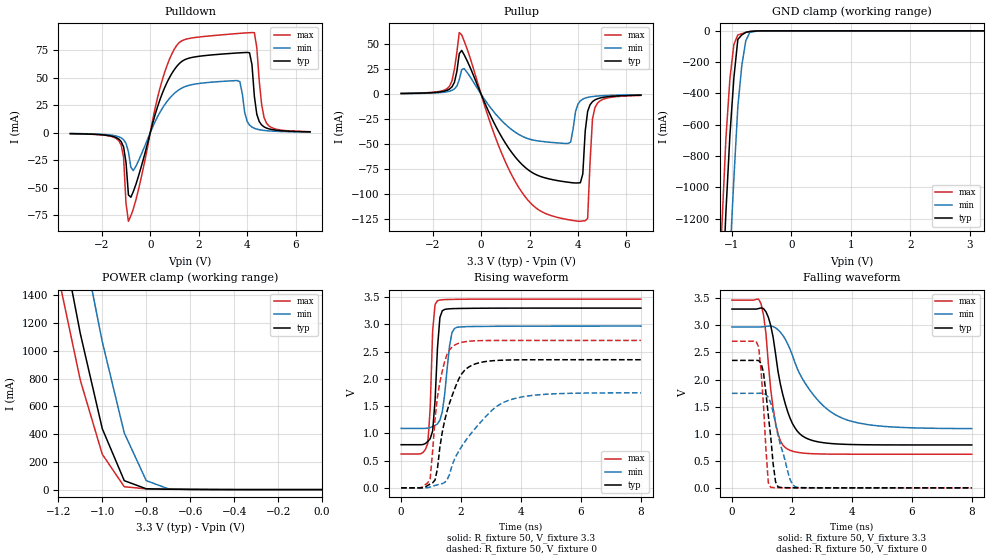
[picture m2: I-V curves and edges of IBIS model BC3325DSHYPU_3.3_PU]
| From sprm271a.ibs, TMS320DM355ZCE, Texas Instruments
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|   Component BC3325DSHYPU
|   Model Cell BC3325DSHYPU_3.3_PU
[Model]   BC3325DSHYPU_3.3_PU
Model_type   I/O
Polarity   Non-Inverting
Enable   Active-Low
Vinl =  1.5
Vinh =  1.8
Cref =  15.0000pF
Rref =  100.0000M
Vref =  0V
Vmeas =  1.65
C_comp   0.972592p   0.9599789p   0.9808023p
[Model Spec]
Vinl   1.5   1.335   1.5825
Vinh   1.8   1.635   1.8825
[Temperature Range]   25   125   -40
[Voltage Range]   3.3   2.97   3.465
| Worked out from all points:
|   slope of the pulldown table from 0 to 0.495 V, typ, clamps not added: 13.9 ohm
|   slope of the pullup table from 0 to 0.495 V, typ, clamps not added: 18.5 ohm
|   GND clamp passes 1 mA (typ) near -0.58 V on its own axis
|   POWER clamp passes 1 mA (typ) near -0.55 V on its own axis
|   rising waveform, R_fixture 50, V_fixture 3.3: 20-80 % time 158ps typ, 222ps min, 119ps max; typ from 0.792 V to 3.3 V
|   rising waveform, R_fixture 50, V_fixture 0: 20-80 % time 596ps typ, 1.31ns min, 352ps max; typ from 0.001 V to 2.35 V
|   falling waveform, R_fixture 50, V_fixture 3.3: 20-80 % time 567ps typ, 1.23ns min, 334ps max; typ from 3.3 V to 0.792 V
|   falling waveform, R_fixture 50, V_fixture 0: 20-80 % time 265ps typ, 467ps min, 185ps max; typ from 2.35 V to 0.001 V
[POWER_clamp]
|   voltage   I(typ)   I(min)   I(max)
-3.3V     22.26A     22.98A     21.87A
-1.2V     1.951A     2.729A     1.539A
-1.167V   1.675A     2.441A     1.289A
-1.133V   1.4A       2.153A     1.039A
-1.1V     1.125A     1.865A     788.5mA
-1.067V   896.1mA    1.599A     610.6mA
-1.033V   667.5mA    1.332A     432.7mA
-1V       438.9mA    1.066A     254.7mA
-900mV    64.51mA    408.4mA    20.8mA
-800mV    5.84mA     64.82mA    5.279mA
-700mV    2.645mA    5.847mA    3.199mA
-11.55fV  455.4pA    9.231nA    227.1pA
[Pulldown]
|   voltage   I(typ)   I(min)   I(max)
-3.3V     -808.1uA   -658.5uA   -838.6uA
-1.3V     -5.711mA   -3.626mA   -7.219mA
-1.1V     -12.9mA    -6.318mA   -22.43mA
-900mV    -56.47mA   -17.38mA   -80.42mA
-700mV    -53.51mA   -34.37mA   -69.3mA
400mV     30.01mA    18.55mA    40.42mA
1.1V      60.43mA    37.7mA     79.59mA
3.7V      72.61mA    46.35mA    90.3mA
4.2V      61.81mA    5.119mA    91.01mA
4.4V      16.79mA    3.291mA    77.1mA
4.8V      4.264mA    1.885mA    8.735mA
6.6V      871.4uA    628.5uA    963.3uA
[Pullup]
|   voltage   I(typ)   I(min)   I(max)
-3.3V     659.6uA    522.1uA    739.6uA
-1.3V     5.126mA    2.966mA    8.081mA
-900mV    40.49mA    14.5mA     61.66mA
-700mV    39.49mA    25.52mA    53.37mA
1.6V      -68.17mA   -40.92mA   -95.13mA
3.6V      -88.21mA   -49.34mA   -125.7mA
4.1V      -88.68mA   -6.718mA   -127.3mA
4.2V      -79.9mA    -4.993mA   -127mA
4.4V      -17.25mA   -3.255mA   -124.4mA
4.6V      -7.503mA   -2.398mA   -24.77mA
4.7V      -5.775mA   -2.116mA   -13.67mA
6.6V      -1.03mA    -644.3uA   -1.277mA
[GND_clamp]
|   voltage   I(typ)   I(min)   I(max)
-3.3V     -22.38A    -23.15A    -21.96A
-1.167V   -1.724A    -2.574A    -1.236A
-1.1V     -1.154A    -1.991A    -682.8mA
-1.033V   -667.2mA   -1.446A    -306.3mA
-966.7mV  -300.6mA   -943.8mA   -87.49mA
-900mV    -54.67mA   -483.6mA   -26.53mA
-833.3mV  -26.4mA    -221.3mA   -17.75mA
-766.7mV  -9.725mA   -63.68mA   -10.41mA
-700mV    -4.652mA   -10.65mA   -4.529mA
-566.7mV  -778.5uA   -1.53mA    -562.3uA
-433.3mV  -131.5uA   -202.2uA   -150.5uA
3.233V    -4.373uA   23.82uA    -20.78uA
[Ramp]
| variable   typ   min   max
dV/dt_f   1.518038/0.5677021n   1.136026/1.235092n   1.721008/0.3340379n
dV/dt_r   1.411463/0.5977116n   1.046785/1.311445n   1.623638/0.3450776n
R_load = 50
[Rising Waveform]
R_fixture = 50
V_fixture = 3.3
V_fixture_min = 2.97
V_fixture_max = 3.465
| time   V(typ)   V(min)   V(max)
|   time   V(typ)   V(min)   V(max)
0s        792.4mV    1.092V     621.4mV
888.9ps   852mV      1.096V     814.8mV
969.7ps   903.9mV    1.107V     1.463V
1.051ns   1.043V     1.126V     2.874V
1.212ns   2.569V     1.175V     3.435V
1.293ns   3.128V     1.243V     3.449V
1.374ns   3.252V     1.399V     3.454V
1.616ns   3.287V     2.612V     3.459V
1.859ns   3.293V     2.947V     3.461V
8ns       3.3V       2.97V      3.465V
[Rising Waveform]
R_fixture = 50
V_fixture = 0
V_fixture_min = 0
V_fixture_max = 0
| time   V(typ)   V(min)   V(max)
|   time   V(typ)   V(min)   V(max)
0s        856.1uV    716.6uV    956.6uV
646.5ps   292uV      502.7uV    3.544mV
969.7ps   71.36mV    13.81mV    170.8mV
1.131ns   144.3mV    44.05mV    1.267V
1.293ns   751.7mV    66.46mV    1.94V
1.535ns   1.416V     151.4mV    2.457V
1.778ns   1.807V     523.1mV    2.618V
2.343ns   2.246V     1.006V     2.696V
3.556ns   2.347V     1.6V       2.706V
8ns       2.353V     1.745V     2.707V
[Falling Waveform]
R_fixture = 50
V_fixture = 3.3
V_fixture_min = 2.97
V_fixture_max = 3.465
| time   V(typ)   V(min)   V(max)
|   time   V(typ)   V(min)   V(max)
0s        3.3V       2.97V      3.465V
969.7ps   3.321V     2.97V      3.398V
1.131ns   3.252V     2.98V      2.86V
1.212ns   3.15V      2.986V     2.302V
1.455ns   2.472V     2.954V     1.195V
1.616ns   1.911V     2.873V     867mV
1.859ns   1.407V     2.656V     714.8mV
2.586ns   892.8mV    1.813V     633.5mV
3.636ns   807.2mV    1.298V     622.3mV
8ns       792.4mV    1.094V     621.4mV
[Falling Waveform]
R_fixture = 50
V_fixture = 0
V_fixture_min = 0
V_fixture_max = 0
| time   V(typ)   V(min)   V(max)
|   time   V(typ)   V(min)   V(max)
0s        2.353V     1.745V     2.707V
888.9ps   2.351V     1.745V     2.601V
969.7ps   2.298V     1.748V     2.166V
1.051ns   2.132V     1.746V     1.536V
1.212ns   1.339V     1.67V      95.23mV
1.293ns   941.8mV    1.569V     10.95mV
1.455ns   110.3mV    1.18V      4.186mV
1.939ns   3.238mV    152.8mV    1.863mV
2.101ns   2.618mV    24.46mV    1.568mV
8ns       856.4uV    726.5uV    956.7uV
